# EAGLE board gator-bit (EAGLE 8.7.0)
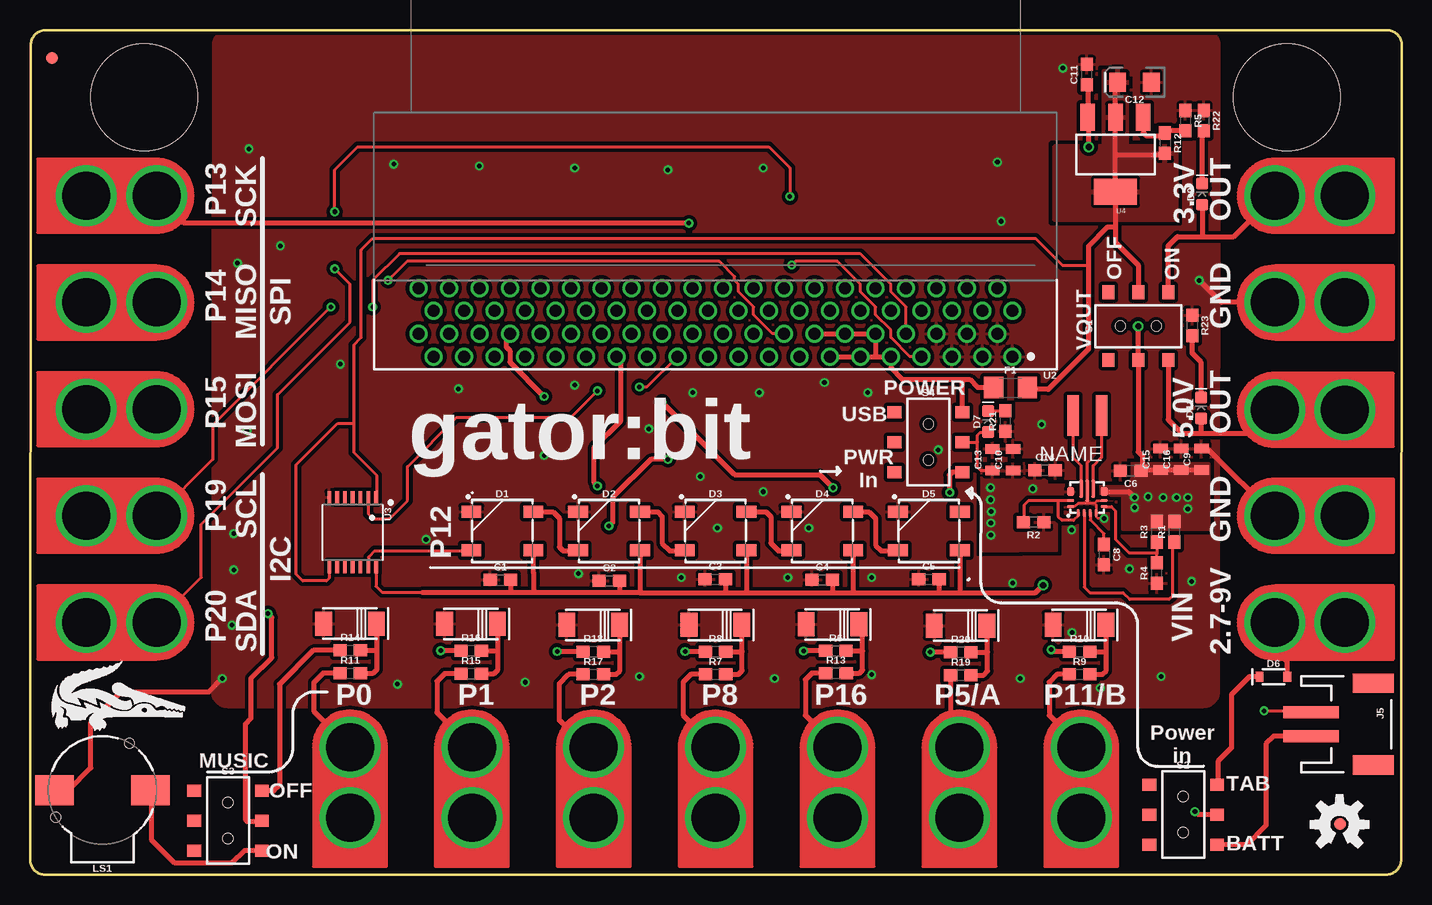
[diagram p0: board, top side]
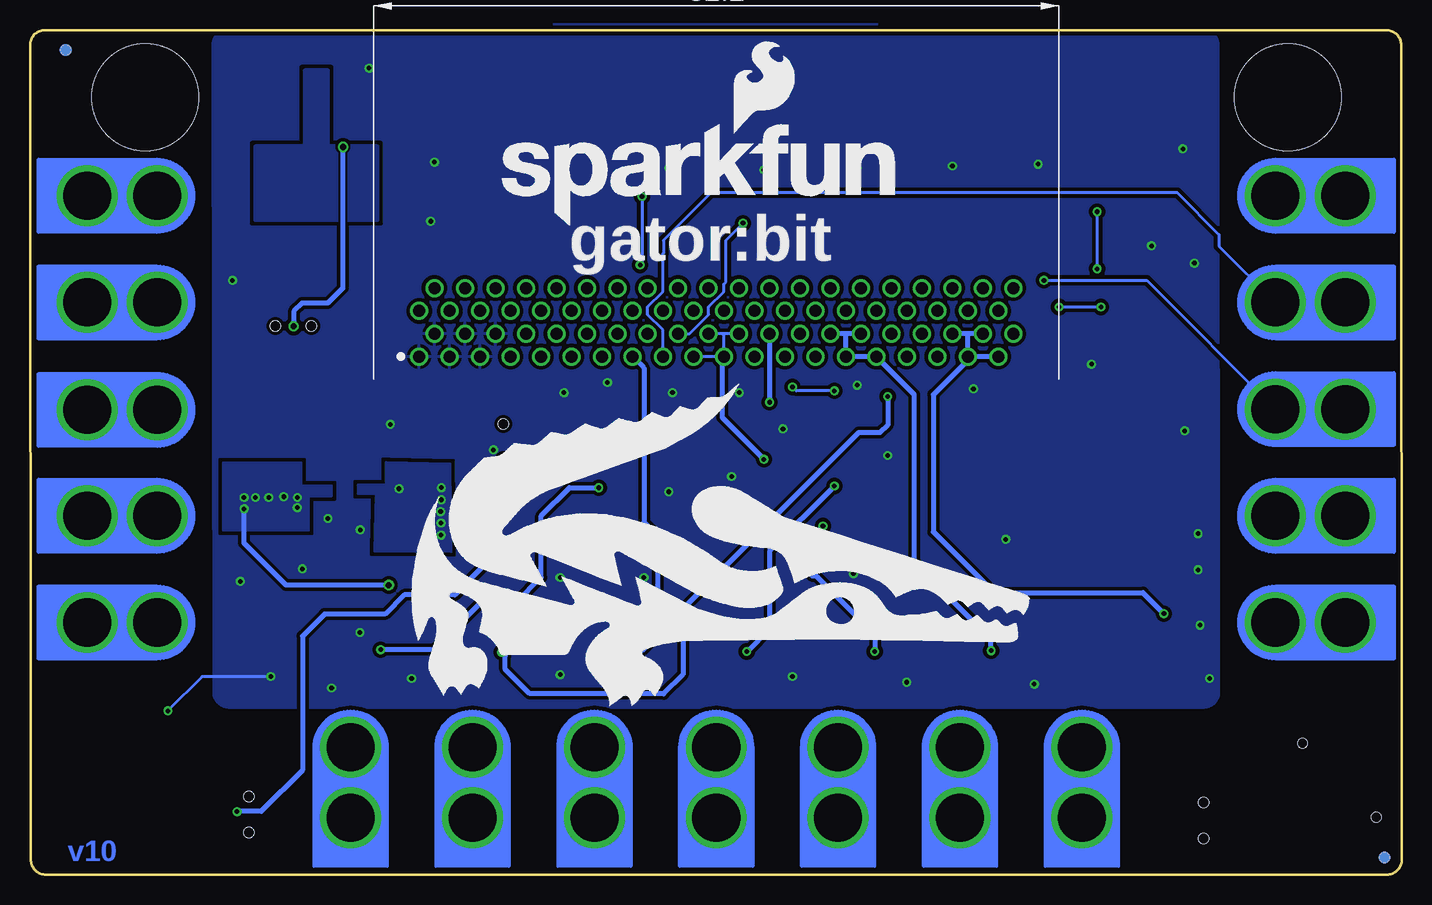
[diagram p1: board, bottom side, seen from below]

Size 114.36 x 70.39 mm. Coordinates in mm from the lower left corner, seen from the top.
Outline: 0.06,69.12 0,1.27 arc90 1.27,0 113.03,0 arc90 114.3,1.27 114.36,69.12 arc90 113.09,70.39 1.33,70.39 arc90 0.06,69.12
Copper layers (1*16): Top 0.035mm / dielectric 1.5mm / Bottom 0.035mm
Design rules "SparkFun-2-layer-TIGHT": minimum track width 7mil, minimum drill 15mil, track to track 7mil, track to pad 7mil, pad to pad 7mil, via to via 7mil, smd to smd 7mil, copper to edge 7mil, drill to drill 7mil, minimum pad ring 7mil, minimum via ring 7mil, stop-mask expansion 4mil, vias tented up to drill 25mil, thermal gap 10mil
Holes 8.89 mm at 9.53,64.77 104.77,64.77

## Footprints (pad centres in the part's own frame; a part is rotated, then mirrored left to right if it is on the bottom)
0603 = smd 1.1 x 1: 1 -0.85,0; 2 0.85,0
0805 = smd 0.8 x 1.2: 1 -0.9,0; 2 0.9,0
EIA3216 = smd 1.4 x 1.6: + 1.4,0; - -1.4,0
WS2812B = smd 1.651 x 1: 1 2.577,-1.6; 2 2.577,1.6; 3 -2.577,1.6; 4 -2.577,-1.6
SOD-323 = smd 0.63 x 0.83: A 1.15,0; C -1.15,0
LED-0603 = smd 1 x 1: A -0.877,0; C 0.877,0
SOD-128 = smd 2 x 1.4: P$1 0,2.5; P$2 0,-1.9
1206 = smd 1.6 x 1.8: 1 -1.4,0; 2 1.4,0
FIDUCIAL-1X2 = smd 1 x 1: 1 0,0
GATOR = drill 4 pad 5.08: P$1 0,-6.096; P$2 0,-0.254
JST-2-SMD = smd 1 x 4.6: 1 -1,-3.7; 2 1,-3.7 | smd 1.6 x 3.4: NC1 -3.4,1.5; NC2 3.4,1.5
XFL4020 = smd 0.965 x 3.404: P$1 1.194,0; P$2 -1.194,0
BUZZER-CCV = smd 3.2 x 2.5: + 4,0; - -4,0 | hole 0.8: -3.9,-2.25; 2.25,3.9
SWITCH_DPDT_SMD_AYZ0202 = smd 1 x 1.15: 1 -2.5,2.825; 2 0,2.825; 3 2.5,2.825; 4 -2.5,-2.825; 5 0,-2.825; 6 2.5,-2.825 | hole 0.85: 1.5,0; -1.5,0
TPS63070RNM = smd 0.6 x 0.25: P$1 0,2.145; P$2 0,1.645; P$3 0,1.145; P$4 0,0.645 | smd 0.25 x 0.6: P$5 0.5,-0.005; P$6 1,-0.005; P$14 1,2.795; P$15 0.5,2.795 | smd 0.75 x 0.6: P$7 1.757,0.006; P$12 1.768,2.794 | smd 1.45 x 0.35: P$9 1.988,0.895; P$11 1.988,1.895 | smd 1.8 x 0.35: P$10 1.812,1.395
MICRO:BIT_RA_PTH = drill 1: A1 -24.765,7.62; A2 -23.495,5.72; A3 -22.225,7.62; A4 -20.955,5.72; A5 -19.685,7.62; A6 -18.415,5.72; A7 -17.145,7.62; A8 -15.875,5.72; A9 -14.605,7.62; A10 -13.335,5.72; A11 -12.065,7.62; A12 -10.795,5.72; A13 -9.525,7.62; A14 -8.255,5.72; A15 -6.985,7.62; A16 -5.715,5.72; A17 -4.445,7.62; A18 -3.175,5.72; A19 -1.905,7.62; A20 -0.635,5.72; A21 0.635,7.62; A22 1.905,5.72; A23 3.175,7.62; A24 4.445,5.72; A25 5.715,7.62; A26 6.985,5.72; A27 8.255,7.62; A28 9.525,5.72; A29 10.795,7.62; A30 12.065,5.72; A31 13.335,7.62; A32 14.605,5.72; A33 15.875,7.62; A34 17.145,5.72; A35 18.415,7.62; A36 19.685,5.72; A37 20.955,7.62; A38 22.225,5.72; A39 23.495,7.62; A40 24.765,5.72; B1 -24.765,3.82; B2 -23.495,1.92; B3 -22.225,3.82; B4 -20.955,1.92; B5 -19.685,3.82; B6 -18.415,1.92; B7 -17.145,3.82; B8 -15.875,1.92; B9 -14.605,3.82; B10 -13.335,1.92; B11 -12.065,3.82; B12 -10.795,1.92; B13 -9.525,3.82; B14 -8.255,1.92; B15 -6.985,3.82; B16 -5.715,1.92; B17 -4.445,3.82; B18 -3.175,1.92; B19 -1.905,3.82; B20 -0.635,1.92; B21 0.635,3.82; B22 1.905,1.92; B23 3.175,3.82; B24 4.445,1.92; B25 5.715,3.82; B26 6.985,1.92; B27 8.255,3.82; B28 9.525,1.92; B29 10.795,3.82; B30 12.065,1.92; B31 13.335,3.82; B32 14.605,1.92; B33 15.875,3.82; B34 17.145,1.92; B35 18.415,3.82; B36 19.685,1.92; B37 20.955,3.82; B38 22.225,1.92; B39 23.495,3.82; B40 24.765,1.92
TSSOP14 = smd 0.305 x 0.991: 1 -1.95,-2.918; 2 -1.3,-2.918; 3 -0.65,-2.918; 4 0,-2.918; 5 0.65,-2.918; 6 1.3,-2.918; 7 1.95,-2.918; 8 1.95,2.918; 9 1.3,2.918; 10 0.65,2.918; 11 0,2.918; 12 -0.65,2.918; 13 -1.3,2.918; 14 -1.95,2.918
SOT223 = smd 1.219 x 2.235: 1 -2.311,-3.099; 2 0,-3.099; 3 2.311,-3.099 | smd 3.6 x 2.2: 4 0,3.099

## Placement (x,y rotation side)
C1  0.1uF  [0603]  39.22,24.56 0 top
C2  0.1uF  [0603]  48.29,24.49 0 top
C3  0.1uF  [0603]  57.13,24.62 0 top
C4  0.1uF  [0603]  66.04,24.56 0 top
C5  0.1uF  [0603]  74.93,24.62 0 top
C6  10uF  [0603]  91.76,33.66 180 top
C8  0.1uF  [0603]  89.53,26.67 270 top
C9  22uF  [0805]  97.65,34.61 90 top
C10  10uF  [0805]  81.95,34.58 90 top
C11  0.1uF  [0603]  88.11,66.67 90 top
C12  10uF  [EIA3216]  92.07,66.04 180 top
C13  10uF  [0805]  80.23,34.58 90 top
C14  10uF  [0603]  84.61,33.72 0 top
C15  22uF  [0805]  94.25,34.61 90 top
C16  22uF  [0805]  95.96,34.61 90 top
D1  WS2812B  [WS2812B]  39.38,28.64 0 top
D2  WS2812B  [WS2812B]  48.27,28.64 0 top
D3  WS2812B  [WS2812B]  57.16,28.64 0 top
D4  WS2812B  [WS2812B]  66.04,28.64 0 top
D5  WS2812B  [WS2812B]  74.93,28.64 0 top
D6  1A/23V/620mV  [SOD-323]  103.66,16.51 0 top
D7  RED  [LED-0603]  79.88,37.76 90 top
D8  3.8V  [SOD-128]  56.83,20.82 270 top
D9  RED  [LED-0603]  97.71,56.71 90 top
D10  3.8V  [SOD-128]  87.19,20.82 270 top
D11  RED  [LED-0603]  97.64,38.89 90 top
D12  3.8V  [SOD-128]  26.38,20.92 270 top
D13  3.8V  [SOD-128]  66.61,20.86 270 top
D15  3.8V  [SOD-128]  36.46,20.89 270 top
D17  3.8V  [SOD-128]  46.65,20.82 270 top
D19  3.8V  [SOD-128]  77.28,20.76 270 top
F1  6V/0.5A  [1206]  81.74,40.59 0 top
FD1  FIDUCIAL1X2  [FIDUCIAL-1X2]  1.47,1.43 0 bottom
FD2  FIDUCIAL1X2  [FIDUCIAL-1X2]  1.81,68.07 0 top
FD3  FIDUCIAL1X2  [FIDUCIAL-1X2]  109.22,4.2 0 top
FD4  FIDUCIAL1X2  [FIDUCIAL-1X2]  111.38,68.7 0 bottom
FRAME1  FRAME-LETTER  [CREATIVE_COMMONS]  not placed on the board
FRAME3  FRAME-LETTER  [CREATIVE_COMMONS]  not placed on the board
J1  GATOR  [GATOR]  103.5,38.73 90 top
J2  GATOR  [GATOR]  103.51,47.69 90 top
J3  GATOR  [GATOR]  103.51,21.02 90 top
J4  GATOR  [GATOR]  103.51,29.91 90 top
J5  [JST-2-SMD]  110.49,12.54 270 top
J6  GATOR  [GATOR]  103.51,56.58 90 top
J7  GATOR  [GATOR]  26.68,10.86 0 top
J8  GATOR  [GATOR]  36.84,10.86 0 top
J9  GATOR  [GATOR]  46.99,10.86 0 top
J10  GATOR  [GATOR]  77.47,10.86 0 top
J11  GATOR  [GATOR]  57.16,10.86 0 top
J12  GATOR  [GATOR]  10.8,56.58 270 top
J13  GATOR  [GATOR]  10.8,47.69 270 top
J14  GATOR  [GATOR]  10.8,38.8 270 top
J15  GATOR  [GATOR]  67.31,10.86 0 top
J16  GATOR  [GATOR]  10.8,29.91 270 top
J17  GATOR  [GATOR]  10.8,21.02 270 top
J18  GATOR  [GATOR]  87.63,10.86 0 top
L1  1.5UH  [XFL4020]  88.14,38.26 180 top
LOGO1  SFE_LOGO_NAME_FLAME.3_INCH  [SFE_LOGO_NAME_FLAME_.3]  75.56,53.98 0 bottom
LOGO2  OSHW-LOGOM  [OSHW-LOGO-M]  109.16,4.19 0 top
LS1  BUZZER-SMD  [BUZZER-CCV]  6.04,7.04 0 top
R1  100k  [0603]  95.42,28.57 90 top
R2  10.2K  [0603]  83.66,29.37 180 top
R3  523k  [0603]  93.94,28.57 90 top
R4  100k  [0603]  93.94,25.13 90 top
R5  390k  [0603]  96.32,62.84 270 top
R6  910  [0603]  67.18,18.64 0 top
R7  604  [0603]  57.15,16.69 0 top
R8  910  [0603]  57.15,18.59 0 top
R9  604  [0603]  87.5,16.69 0 top
R10  910  [0603]  87.5,18.59 0 top
R11  604  [0603]  26.7,16.79 0 top
R12  240  [0603]  94.61,60.96 270 top
R13  604  [0603]  67.19,16.8 0 top
R14  910  [0603]  26.7,18.69 0 top
R15  604  [0603]  36.78,16.76 0 top
R16  910  [0603]  36.78,18.67 0 top
R17  604  [0603]  46.96,16.69 0 top
R18  910  [0603]  46.96,18.59 0 top
R19  604  [0603]  77.6,16.64 0 top
R20  910  [0603]  77.6,18.54 0 top
R21  1k  [0603]  81.32,37.81 90 top
R22  1k  [0603]  97.84,62.84 270 top
R23  1k  [0603]  96.88,45.77 270 top
S1  [SWITCH_DPDT_SMD_AYZ0202]  92.39,45.72 0 top
S2  [SWITCH_DPDT_SMD_AYZ0202]  96.13,5 270 top
S3  [SWITCH_DPDT_SMD_AYZ0202]  16.52,4.5 270 top
S4  [SWITCH_DPDT_SMD_AYZ0202]  74.89,36.04 270 top
U1  TPS63070  [TPS63070RNM]  89.53,30.16 90 top
U2  micro:bit  [MICRO:BIT_RA_PTH]  57.15,50.8 180 top
U3  TXB0104  [TSSOP14]  26.9,28.52 180 top
U4  ADJ REG 1.5A  [SOT223]  90.49,60.01 180 top
U$4  [ORDERING_INSTRUCTIONS]  not placed on the board

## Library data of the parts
C1-C5 C8 C11 = SparkFun-Capacitors; PROD_ID: CAP-00810
C6 C14 = SparkFun-Capacitors; PROD_ID: CAP-11015
C9 C15 C16 = SparkFun-Capacitors; PROD_ID: CAP-08402
C10 C13 = SparkFun-Capacitors; PROD_ID: CAP-11330
C12 = SparkFun-Capacitors; PROD_ID: CAP-00811
D1-D5 = SparkFun-LED; PROD_ID: DIO-12503
D6 = SparkFun-DiscreteSemi; PROD_ID: DIO-11623
D7 D9 D11 = SparkFun-LED; PROD_ID: DIO-00819
D8 D10 D12 D13 D15 D17 D19 = PDZVTR36BCT; PROD_ID: DIO-13895; TECHNOLOGIES: Zener Diode 3.8V 1W ±5.26% Surface Mount PMDTM
F1 = SparkFun-Fuses; PROD_ID: RES-08585
FD1-FD4 FRAME1 FRAME3 LOGO1 LOGO2 U$4 = SparkFun-Aesthetics
J1-J4 J6-J18 = TAB
J5 = SparkFun-Connectors; PROD_ID: CONN-11443
L1 = SparkFun-Coils; PROD_ID: NDUC-13855
LS1 = SparkFun-Electromechanical; PROD_ID: COMP-08568
R1 R4 = SparkFun-Resistors; PROD_ID: RES-07828
R2 = SparkFun-Resistors; PROD_ID: RES-13856
R3 = SparkFun-Resistors; PROD_ID: RES-13864
R5 = SparkFun-Resistors; PROD_ID: RES-12024
R6 R8 R10 R14 R16 R18 R20 = SparkFun-Resistors; PROD_ID: RES-13860
R7 R9 R11 R13 R15 R17 R19 = SparkFun-Resistors; PROD_ID: RES-13857
R12 = SparkFun-Resistors; PROD_ID: RES-07849
R21-R23 = SparkFun-Resistors; PROD_ID: RES-07856
S1 = SparkFun-Switches; PROD_ID: SWCH-08179; SF_SKU: COM-00597
S2-S4 = SparkFun-Switches; PROD_ID: SWCH-08179; SF_ID: COM-00597
U1 = SparkFun-IC-Power; PROD_ID: IC-13858
U2 = Micro_Bit_Parts; PROD_ID: CONN-13452
U3 = SparkFun-IC-Comms; PROD_ID: IC-13929
U4 = SparkFun-IC-Power; PROD_ID: VREG-12029

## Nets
3.3V: C12.+ F1.2 R12.2 S1.2 U3.1 U3.8 U4.2 U4.4
5V: C1.2 C2.2 C3.2 C4.2 C5.2 C6.1 C9.1 C11.1 C15.1 C16.1 D1.1 D2.1 D3.1 D4.1 D5.1 R1.2 R3.2 S1.5 U1.P$7 U3.14 U4.3
GND: C1.1 C2.1 C3.1 C4.1 C5.1 C6.2 C8.2 C9.2 C10.2 C11.2 C12.- C13.2 C14.2 C15.2 C16.2 D1.3 D2.3 D3.3 D4.3 D5.3 D8.P$2 D10.P$2 D12.P$2 D13.P$2 D15.P$2 D17.P$2 D19.P$2 J2.P$1 J2.P$2 J4.P$1 J4.P$2 J5.1 LS1.- R4.1 R5.1 R21.1 R22.1 R23.1 U1.P$4 U1.P$6 U1.P$10 U1.P$15 U2.A1 U2.A2 U2.A3 U2.A4 U2.A5 U2.A6 U3.7
MBIN: F1.1 S4.1 U2.A9 U2.A10 U2.A11 U2.A12 U2.A13 U2.A14
N$2: L1.P$1 U1.P$11
N$3: LS1.+ S3.3
N$4: D1.2 D2.4
N$5: D2.2 D3.4
N$6: D3.2 D4.4
N$7: D4.2 D5.4
N$8: L1.P$2 U1.P$9
N$9: D7.C R21.2
N$11: R3.1 R4.2 U1.P$5
N$12: C8.1 U1.P$3
N$13: R2.2 U1.P$1 U1.P$14
N$14: R1.1 U1.P$2
N$16: R5.2 R12.1 U4.1
N$20: D6.C S2.1
N$23: D9.C R22.2
N$24: D11.C R23.2
P0: S3.2 U2.A36 U2.A37 U2.A38 U2.A39
P0+: J7.P$1 J7.P$2 R11.1
P1: R16.1 U2.A28 U2.A29 U2.A30 U2.A31
P1+: J8.P$1 J8.P$2 R15.1
P2: R18.1 U2.A19 U2.A20 U2.A21 U2.A22
P2+: J9.P$1 J9.P$2 R17.1
P5: R20.1 U2.A34
P5+: J10.P$1 J10.P$2 R19.1
P8: R8.1 U2.A27
P8+: J11.P$1 J11.P$2 R7.1
P11: R10.1 U2.A24
P11+: J18.P$1 J18.P$2 R9.1
P12: D1.4 U3.13
P12LL: U2.A23 U3.2
P13: J12.P$1 J12.P$2 U2.A18
P14: J13.P$1 J13.P$2 U2.A17
P15: J14.P$1 J14.P$2 U2.A16
P16: R6.1 U2.A15
P16+: J15.P$1 J15.P$2 R13.1
P19: J16.P$1 J16.P$2 U2.A8
P20: J17.P$1 J17.P$2 U2.A7
PD: R14.1 S3.1
PP0: D12.P$1 R11.2 R14.2
PP1: D15.P$1 R15.2 R16.2
PP2: D17.P$1 R17.2 R18.2
PP5: D19.P$1 R19.2 R20.2
PP8: D8.P$1 R7.2 R8.2
PP11: D10.P$1 R9.2 R10.2
PP16: D13.P$1 R6.2 R13.2
V_BATT: J5.2 S2.3
VIN: C10.1 C13.1 C14.1 D7.A R2.1 S4.2 U1.P$12
VIN_TAB: D6.A J3.P$1 J3.P$2
VOUT3.3: D9.A J6.P$1 J6.P$2 S1.3
VOUT5.0: D11.A J1.P$1 J1.P$2 S1.6
VSUPPLY: S2.2 S4.3

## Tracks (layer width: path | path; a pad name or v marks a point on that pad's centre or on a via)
3.3V
  Top 0.254: 88.26,50.8 86.04,50.8 83.82,53.02 28.57,53.02 27.62,52.07 27.62,44.77 26.99,44.13 26.99,37.72 | 26.99,37.72 26.99,35.19 28.88,33.3 28.88,31.47 U3.1 | U3.8 24.95,24.72 24.71,24.49 22.73,24.49 22.2,25.02 22.2,34.16 25.65,37.62 26.89,37.62 26.99,37.72
  Top 0.406: 90.49,53.98 U4.4 90.49,60.01 | 90.49,53.98 90.49,52.7 92.39,50.8 S1.2 | 90.49,53.98 89.85,53.98 88.26,52.39 88.26,50.8 88.26,43.81 84.89,40.44 83.29,40.44 F1.2 | C12.+ 90.49,65.85 U4.2 90.49,60.01 | 90.49,60.01 94.51,60.01 R12.2
  pour Top (isolate 0.305): 89.53,66.99 89.53,60.64 85.41,60.64 85.41,54.61 95.57,54.61 95.57,60.64 91.44,60.64 91.44,66.99
5V  (via drill 0.38, 0.51)
  Top 0.254: U3.14 28.85,24.03 29.36,23.52 33.38,23.52 33.4,23.5
  Top 0.406: C11.1 88.18,65.75 U4.3 88.26,63.02 v88.26,60.64 | 50.8,23.5 58.1,23.5 | 58.1,23.5 59.69,23.5 | 59.69,23.5 66.99,23.5 | 66.99,23.5 68.58,23.5 | 68.58,23.5 75.88,23.5 | 75.88,23.5 77.47,23.5 | 77.47,23.5 83.82,23.5 v84.45,24.13 | D1.1 41.95,25.18 41.96,25.18 41.96,23.5 | D2.1 50.84,23.54 50.8,23.5 | 58.1,23.5 57.98,23.62 C3.2 | D3.1 59.73,23.54 59.69,23.5 | C4.2 66.89,23.59 66.99,23.5 | D4.1 68.62,23.54 68.58,23.5 | C5.2 75.78,23.59 75.88,23.5 | D5.1 77.51,23.54 77.47,23.5 | C9.1 C16.1 C15.1 92.66,33.71 C6.1 92.71,33.76 92.71,34.92 92.39,35.24 S1.5 92.39,45.69 v92.38,45.71 | U1.P$7 91.59,31.92 v92.07,31.43 | 50.8,23.5 49.1,23.5 | 49.1,23.5 41.96,23.5 | 41.96,23.5 40.13,23.5 | 40.13,23.5 33.4,23.5 32.7,23.5 | C1.2 40.07,23.55 40.13,23.5 | C2.2 49.14,23.54 49.1,23.5
  Bottom 0.406: v84.45,24.13 93.03,24.13 96.52,27.62 v96.52,30.48 | v88.26,60.64 88.26,48.9 89.53,47.62 91.69,47.62 92.38,46.93 v92.38,45.71
  other vias: 95.57,31.43 94.46,31.43 93.21,31.5 96.52,31.43 92.09,30.58
  pour Top (isolate 0.305, no thermals): 89.22,32.38 91.76,32.38 91.76,34.29 98.27,34.29 98.27,28.73 91.12,28.73 91.12,31.59 89.22,31.59
  pour Bottom: 91.12,28.73 91.12,31.59 89.22,31.59 89.22,32.38 91.76,32.38 91.76,34.29 98.27,34.29 98.27,28.73
GND  (via drill 0.38)
  Top 0.203: 88.73,30.93 88.96,31.16 U1.P$6 | 88.73,30.93 88.89,30.78 U1.P$4 88.89,29.86 88.9,29.84 88.9,29.81 89.02,29.69 v89.53,29.69 | U1.P$15 87.02,30.66 87.05,30.68 87.12,30.68 87.38,30.94 88.73,30.94 88.73,30.93
  Top 0.254: U1.P$10 88.14,34.32 88.26,34.45 | v102.87,13.65 106.04,13.65 106.36,13.34 106.58,13.34 J5.1
  Top 0.406: 97.63,49.37 99.32,47.69 J2.P$2 J2.P$1 109.54,47.75 | LS1.- 3.23,7.04 5.08,8.89 5.08,12.7 7.62,15.24 14.92,15.24 v16.03,16.35 | C9.2 98.16,35.51 J4.P$2 J4.P$1 109.54,29.97
  Bottom 0.254: v94.3,16.51 100.01,16.51 v102.87,13.65
  other vias: 97.47,49.53 16.99,25.4 16.83,20.8 30.64,15.88 41.27,16.03 50.8,16.51 62.07,16.35 57.31,28.89 16.99,28.42 18.26,60.48 17.3,50.96 20.87,52.41 42.86,34.92 37.47,59.05 45.4,58.9 53.18,58.74 69.85,40.16 61.12,58.9 45.4,40.8 51.59,37.15 61.12,31.91 84.33,37.53 18.1,36.99 80.64,59.37 86.11,67.21 80.96,54.45 86.84,28.73 75.72,35.4 81.91,24.29 91.65,25.49 70.17,16.67 82.55,16.35 55.88,33.18 64.93,28.89 30.32,59.21 25.88,42.55 60.8,40.16 55.24,40.16 86.87,20.18 96.84,24.45 89.22,15.56 35.72,40.48 66.23,41.01 70.17,24.77 63.18,24.77 54.29,24.77 45.72,25.08 33.02,27.94
  pour Top (isolate 0.305, rank 2): 15.24,15.24 15.3,69.12 arc-90 16.57,70.39 97.85,70.39 arc-90 99.12,69.12 99.06,15.24 arc-90 97.79,13.97 16.51,13.97 arc-90
  pour Bottom (isolate 0.305, rank 2): 15.24,15.24 15.3,69.12 arc-90 16.57,70.39 arc-3 97.85,70.39 arc-90 99.12,69.12 99.06,15.24 arc-90 97.79,13.97 16.51,13.97 arc-90
MBIN
  Top 0.406: U2.A13 U2.A11 70.48,43.18 | 70.48,43.18 U2.A9 71.75,42.23 72.71,41.27 77.9,41.27 | U2.A14 U2.A12 U2.A10 70.48,43.18 | S4.1 77.72,41.09 77.9,41.27 | 77.9,41.27 78.33,41.27 78.99,40.62 80.31,40.62 F1.1
N$2
  Top 0.254: U1.P$11 87.64,34.09 86.93,34.8 86.94,34.81 L1.P$1
N$3
  Top 0.406: S3.3 17.88,2 16.83,0.95 12.06,0.95 10.16,2.86 10.16,6.92 LS1.+
N$4
  Top 0.406: D1.2 43.58,30.23 44.13,29.69 44.13,27.3 44.45,26.99 46.04,26.99 46.2,26.83 45.89,26.83 D2.4
N$5
  Top 0.406: D2.2 52.31,30.23 52.7,29.84 52.7,27.62 53.34,26.99 54.53,26.99 D3.4
N$6
  Top 0.406: D3.2 61.36,30.23 61.75,29.84 61.75,27.62 62.39,26.99 63.42,26.99 D4.4
N$7
  Top 0.406: D4.2 69.94,30.23 70.48,29.69 70.48,27.46 70.96,26.99 72.31,26.99 D5.4
N$8
  Top 0.254: U1.P$9 88.64,34.09 89.33,34.78 L1.P$2
N$9
  Top 0.254: D7.C 81.31,38.64 R21.2
N$11
  Top 0.254: U1.P$5 90.15,30.66 90.49,30.32 90.49,27.94 91.6,26.83 93.87,26.83 93.95,26.75 | R3.1 93.95,27.71 93.95,26.75 | R4.2 93.94,26.73 93.95,26.75
N$12
  Top 0.254: U1.P$3 88.39,29.56 89.53,28.42 C8.1
N$13
  Top 0.254: U1.P$1 87.39,29.92 86.99,29.53 86.04,29.53 85.72,29.84 85.72,31.16 | U1.P$14 85.72,31.16 | 85.72,31.16 83.23,31.16 82.87,30.8 82.87,29.43 R2.2
N$14
  Top 0.254: U1.P$2 87.89,23.96 88.36,23.5 91.12,23.5 91.68,22.94 94.94,22.94 95.26,23.25 95.26,27.57 R1.1
N$16
  Top 0.406: U4.1 92.8,61.82 93.03,61.59 94.4,61.59 R12.1 94.79,61.99 R5.2
N$20
  Top 0.406: D6.C 101.65,16.51 100.15,15.01 100.15,10.57 99.03,9.45 99.03,7.59 S2.1
N$22
  pour Bottom: 89.53,66.99 91.44,66.99 91.44,60.64 95.57,60.64 95.57,54.61 85.41,54.61 85.41,60.64 89.53,60.64
N$23
  Top 0.406: D9.C 97.71,61.86 R22.2
N$24
  Top 0.406: D11.C 97.64,42.7 96.88,43.46 R23.2
P0  (via drill 0.38)
  Top 0.254: v19.84,21.75 19.84,21.59
  Top 0.406: v19.84,21.75 20.16,21.43 20.16,18.1 18.41,16.35 18.41,13.02 17.94,12.54 17.94,4.6 18.1,4.45 19.28,4.45 S3.2
  Bottom 0.406: U2.A38 36.19,45.08 | 36.19,45.08 U2.A36 | U2.A37 36.19,45.08 | U2.A39 U2.A37 | U2.A37 36.19,42.86 39.05,40.01 39.05,28.57 33.97,23.5 21.59,23.5 v19.84,21.75
P0+
  Top 0.406: J7.P$1 J7.P$2 23.65,13.63 23.65,16 24.43,16.79 R11.1
P1  (via drill 0.38)
  Top 0.406: R16.1 v34.24,18.67
  Bottom 0.406: U2.A30 46.35,45.08 | 46.35,45.08 U2.A28 | 46.35,45.08 U2.A29 U2.A31 40.64,40.01 40.64,26.02 34.24,19.62 v34.24,18.67
P1+
  Top 0.406: J8.P$1 J8.P$2 33.92,13.51 33.92,16.13 34.56,16.76 R15.1
P2  (via drill 0.38)
  Top 0.406: R18.1 v43.95,18.59 | v53.18,34.61 51.75,34.61 48.58,31.43 48.58,29.37 v48.26,29.05
  Bottom 0.254: U2.A22 56.67,45.08 | 56.67,45.08 U2.A20 | 56.67,43.18 U2.A19 | U2.A21 56.51,44.92 56.67,45.08
  Bottom 0.406: U2.A21 56.67,43.18 56.67,38.1 v53.18,34.61 | v48.26,29.05 49.21,28.1 49.21,24.92 48.85,24.92 43.92,19.99 43.92,18.62 v43.95,18.59
P2+
  Top 0.406: J9.P$1 J9.P$2 46.87,10.48 46.51,10.48 44.13,12.86 44.13,15.92 44.9,16.69 R17.1
P5  (via drill 0.38)
  Top 0.406: v42.86,39.85 40,42.7 40,43.66 39.69,43.97 39.69,44.61 40,44.93 U2.A34 | R20.1 v75.06,18.54
  Bottom 0.406: v75.06,18.54 74.74,18.22 74.74,17.11 72.71,15.08 65.88,15.08 65.86,15.06 61.54,15.06 59.94,16.66 59.94,22.17 45.29,36.83 43.5,36.83 42.86,37.47 v42.86,39.85
P5+
  Top 0.406: J10.P$1 J10.P$2 76.75,11.33 R19.1
P8  (via drill 0.38)
  Top 0.406: U2.A27 49.21,42.86 49.21,37.78 46.99,35.56 46.99,32.7 v47.31,32.38 | R8.1 v54.61,18.59
  Bottom 0.406: v54.61,18.59 52.7,20.5 52.7,26.99 v47.31,32.38
P8+
  Top 0.406: J11.P$1 J11.P$2 54.45,13.3 54.45,16.05 55.09,16.69 R7.1
P11  (via drill 0.38)
  Top 0.406: v52.7,39.37 58.74,33.34 65.85,33.34 v66.94,32.24 | R10.1 85.28,18.59 v85.12,18.75
  Bottom 0.406: U2.A24 v52.7,39.37 | v66.94,32.24 66.95,32.26 69.39,32.26 71.75,29.9 71.75,24.77 73.82,22.7 76.76,22.7 80.72,18.75 v85.12,18.75
P11+
  Top 0.406: J18.P$1 J18.P$2 84.96,13.27 84.96,16.05 85.6,16.69 R9.1
P12
  Top 0.254: D1.4 36.75,26.99 28.74,26.99 28.22,26.47 28.22,25.63 U3.13
P12LL  (via drill 0.38)
  Top 0.254: v47.31,40.32 45.08,38.1 35.56,38.1 31.47,34.01 31.47,31.17 29.97,29.67 28.6,29.67 28.2,30.07 U3.2 | v50.8,40.64 51.43,40.64 U2.A23
  Bottom 0.254: v47.31,40.32 50.48,40.32 v50.8,40.64
P13  (via drill 0.38)
  Top 0.406: v54.93,54.29 12.83,54.29 J12.P$2
  Bottom 0.254: U2.A18 59.38,45.08 57.78,46.67 57.78,47.31 56.51,48.58 56.51,49.21 56.36,49.37 56.36,52.86 v54.93,54.29
  Bottom 0.406: J12.P$1 J12.P$2
P14
  Bottom 0.254: U2.A17 61.59,45.4 62.86,46.67 62.86,47.31 61.59,48.58 61.59,51.75 61.57,51.78 61.57,52.86 57.59,56.83 18.73,56.83 15.24,53.34 15.24,52.38 J13.P$2
  Bottom 0.406: J13.P$1 J13.P$2
P15  (via drill 0.38)
  Top 0.254: U2.A16 61.91,45.09 60.32,46.67 60.32,47.31 59.05,48.58 59.05,49.21 58.74,49.53 58.74,49.85 57.47,51.12 31.43,51.12 v29.84,49.53
  Bottom 0.254: v29.84,49.53 21.27,49.53 21.27,49.52 J14.P$2
  Bottom 0.406: J14.P$1 J14.P$2
P16  (via drill 0.38)
  Top 0.406: R6.1 v64.48,18.64
  Bottom 0.406: U2.A15 63.18,42.23 63.18,29.37 62.07,28.26 62.07,19.95 63.35,18.67 64.46,18.67 v64.48,18.64
P16+
  Top 0.406: J15.P$1 J15.P$2 64.64,13.27 64.64,16.26 65.18,16.8 R13.1
P19  (via drill 0.38)
  Top 0.254: U2.A8 73.02,47.31 71.75,48.58 71.75,49.21 69.21,51.75 30.8,51.75 28.57,49.53 v28.57,47.31 | v25.08,47.31 15.24,37.47 15.24,34.6 J16.P$2
  Top 0.406: J16.P$1 J16.P$2
  Bottom 0.254: v28.57,47.31 v25.08,47.31
P20  (via drill 0.38)
  Top 0.254: v25.4,50.48 26.67,49.21 26.67,46.04 20.64,40.01 20.64,35.56 14.29,29.21 14.29,24.77 J17.P$2 | v63.5,50.8 63.82,51.12 67.31,51.12 69.21,49.21 69.21,48.58 70.48,47.31 70.48,46.67 71.75,45.4 71.75,44.77 73.34,43.18 U2.A7 | v25.4,55.24 25.4,58.74 27.3,60.64 61.59,60.64 63.34,58.9 v63.34,56.52
  Bottom 0.254: v25.4,50.48 v25.4,55.24 | v63.34,56.52 63.34,50.96 v63.5,50.8
  Bottom 0.406: J17.P$1 9.78,21.02 10.16,20.64 10.17,20.64 J17.P$2
PD
  Top 0.406: S3.1 19.36,6.99 20.32,6.99 20.8,7.46 20.8,15.88 23.62,18.69 R14.1
PP0
  Top 0.406: R11.2 28.6,16.79 28.92,17.11 28.92,18.69 | 28.92,18.69 28.92,20.88 D12.P$1 | R14.2 28.92,18.69
PP1
  Top 0.406: R15.2 38.68,16.76 39,17.08 39,18.67 | 39,18.67 39,20.85 D15.P$1 | R16.2 39,18.67
PP2
  Top 0.406: R17.2 48.87,16.69 49.19,17 49.19,18.59 | 49.19,18.59 49.19,20.77 D17.P$1 | R18.2 49.19,18.59
PP5
  Top 0.406: R19.2 79.5,16.64 79.82,16.95 79.82,18.54 | 79.82,18.54 79.82,20.72 D19.P$1 | R20.2 79.82,18.54
PP8
  Top 0.406: R7.2 59.05,16.69 59.37,17 59.37,18.59 | 59.37,18.59 59.37,20.77 D8.P$1 | R8.2 59.37,18.59
PP11
  Top 0.406: R9.2 89.41,16.69 89.73,17 89.73,18.59 | 89.73,18.59 89.73,20.77 D10.P$1 | R10.2 89.73,18.59
PP16
  Top 0.406: R13.2 69.15,16.8 69.41,17.06 69.41,18.64 | 69.41,18.64 69.41,20.56 D13.P$1 | R6.2 69.41,18.64
V_BATT
  Top 0.406: J5.2 103.67,11.54 103.02,10.9 103.02,4.12 101.42,2.52 98.96,2.52 S2.3
VIN  (via drill 0.38)
  Top 0.254: 86.74,32.1 86.91,31.93 86.74,31.76 86.74,31.68 | 79.79,36.8 D7.A 79.86,36.86 79.22,36.86 78.99,36.64 78.99,36.04 | 78.99,36.04 78.99,33.94 79.26,33.68 C13.1 | S4.2 78.99,36.04
  other vias: 80.07,32.26 80.07,31.24 80.14,30.26 80.11,29.31 80.11,28.29 83.6,32.16
  pour Top (isolate 0.305): 79.34,34.23 84.68,34.32 84.71,32.48 84.93,32.48 86.99,32.51 86.99,31.59 86.04,31.59 85.57,31.11 85.57,26.99 79.34,26.92
  pour Bottom (isolate 0.305): 79.33,34.26 84.68,34.35 84.68,32.51 86.99,32.51 86.99,31.75 85.5,31.73 85.61,26.95 79.26,26.92
VIN_TAB
  Top 0.406: J3.P$1 J3.P$2 103.76,18.79 104.77,17.78 104.77,16.55 D6.A
VOUT3.3
  Top 0.254: J6.P$2 J6.P$1
  Top 0.406: S1.3 94.89,52.4 95.66,53.16 97.79,53.16 | 103.51,56.83 J6.P$2 | J6.P$2 103.76,53.92 | 97.79,53.16 100.35,53.16 J6.P$2 | D9.A 97.71,53.24 97.79,53.16
VOUT5.0
  Top 0.406: S1.6 94.89,37.92 96.01,36.8 97.61,36.8 | J1.P$2 J1.P$1 | J1.P$2 103.76,36.45 | D11.A 97.62,38.02 97.62,36.82 97.61,36.8 | 97.61,36.8 101.83,36.8 J1.P$2
VSUPPLY  (via drill 0.38)
  Top 0.406: v76.68,31.85 76.63,31.9 76.63,33.3 76.89,33.55 76.9,33.54 S4.3 | S2.2 97.36,5 v97.1,5.26
  Bottom 0.406: v76.68,31.85 76.66,31.83 76.66,25.6 78.94,23.32 83.16,23.32 84.76,21.72 89.81,21.72 91.64,19.89 91.64,8.71 95.07,5.28 97.08,5.28 v97.1,5.26

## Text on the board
Bottom: v10
tPlace: P13 | SCK | 3.3V | OUT | MISO | P14 | SPI | OFF | ON | GND | VOUT | P15 | MOSI | POWER | USB | OUT | 5.0V | gator:bit | PWR / In | P19 | SCL | I2C | GND | P12 | 2.7-9V | P20 | SDA | VIN | P0 | P1 | P2 | P8 | P16 | P5/A | P11/B | Power / in | MUSIC | OFF | TAB | ON | BATT
bPlace: gator:bit
Measures: * All dimensions / are in inches
tDocu: Mary West | Solder Mask: Black Gloss

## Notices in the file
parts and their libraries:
SparkFun-Aesthetics: Licensing: Creative Commons ShareAlike 4.0 International - https://creativecommons.org/licenses/by-sa/4.0
SparkFun-Aesthetics: Released under the Creative Commons Attribution Share-Alike 4.0 License
SparkFun-Aesthetics: https://creativecommons.org/licenses/by-sa/4.0
